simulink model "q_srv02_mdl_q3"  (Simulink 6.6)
settings: Solver=ode1  StartTime=0.0  StopTime=0.5  FixedStep=0.002  RelTol=1e-3  AbsTol=1e-6
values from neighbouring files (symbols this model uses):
  K = Am / Beq_v    [d_model_param.m]    (also in setup_srv02_exp01_mdl.m = 1)
  K_ENC = 0    [config_srv02.m]
  K_POT = -(352 * pi / 180 / 10)    (= -0.614355896702)    [config_srv02.m]
  K_TACH = -(1000 * 2 * pi / 60 / 1.5 / Kg)    [config_srv02.m]
  VMAX_DAC = 10    [setup_srv02_exp01_mdl.m]    (also in setup_srv02_exp02_pos.m; setup_srv02_exp03_spd.m)
  wcf_e = 2 * pi * 25.0    (= 157.079632679)    [setup_srv02_exp01_mdl.m]    (also in setup_srv02_exp02_pos.m = 314.159265359; setup_srv02_exp03_spd.m = 395.840674352)
  zetaf_e = 0.9    [setup_srv02_exp01_mdl.m]    (also in setup_srv02_exp02_pos.m; setup_srv02_exp03_spd.m)
undefined symbols (not defined in the file or in its folder): HIL, IMAX_UPM, qc_get_step_size
libraries: quarc_library x5

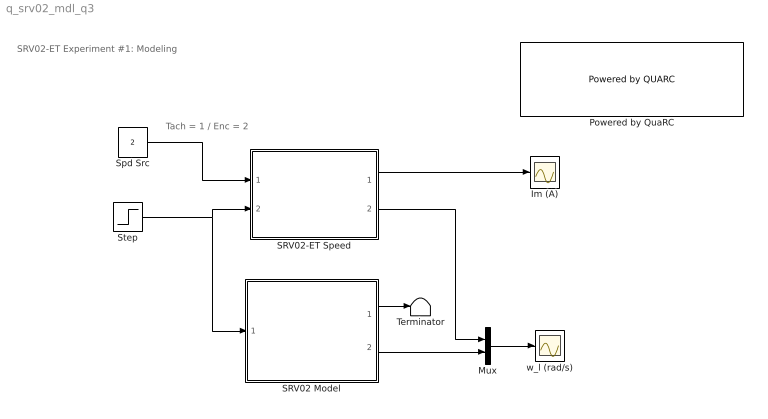
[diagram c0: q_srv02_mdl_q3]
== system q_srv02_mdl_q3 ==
  note: SRV02-ET Experiment #1: Modeling
  note: Tach = 1 / Enc = 2
  Im (A) : Scope
  Mux : Mux  Inputs=2
  Powered by QuaRC : quarc_library/Logos/Powered by QUARC  SystemSampleTime=-1
  SRV02 Model : Subsystem
  SRV02-ET Speed : Subsystem
  Spd Src : Constant  Value=2
  Step : Step  Time=0.1  SampleTime=0
  Terminator : Terminator
  w_l (rad/s) : Scope
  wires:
  Mux/1 -> w_l (rad/s)/1
  SRV02-ET Speed/1(Im (A)) -> Im (A)/1
  SRV02 Model/2(omega_l (rad/s)) -> Mux/2
  SRV02-ET Speed/2(omega_l (rad/s)) -> Mux/1
  SRV02 Model/1(theta_l (rad)) -> Terminator/1
  Spd Src/1 -> SRV02-ET Speed/1(spd src)
  Step/1 -> SRV02-ET Speed/2(I_ref (A)), SRV02 Model/1(I_ref (A))

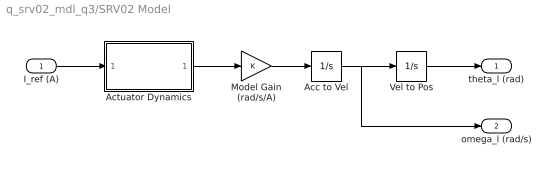
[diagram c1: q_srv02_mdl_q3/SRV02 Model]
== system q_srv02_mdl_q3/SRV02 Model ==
  I_ref (A) : Inport
  Acc to Vel : Integrator
  Actuator Dynamics : Subsystem
  Model Gain (rad/s/A) : Gain  Gain=K
  Vel to Pos : Integrator
  theta_l (rad) : Outport
  omega_l (rad/s) : Outport  Port=2
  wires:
  I_ref (A)/1 -> Actuator Dynamics/1(I_ref (A))
  Acc to Vel/1 -> omega_l (rad/s)/1, Vel to Pos/1
  Actuator Dynamics/1(Im (A)) -> Model Gain (rad/s/A)/1
  Model Gain (rad/s/A)/1 -> Acc to Vel/1
  Vel to Pos/1 -> theta_l (rad)/1

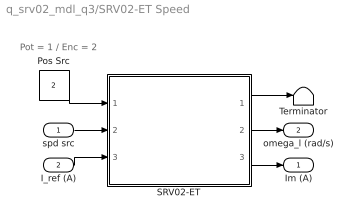
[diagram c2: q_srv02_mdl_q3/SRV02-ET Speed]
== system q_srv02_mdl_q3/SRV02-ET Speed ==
  note: Pot = 1 / Enc = 2
  spd src : Inport
  I_ref (A) : Inport  Port=2
  Pos Src : Constant  Value=2
  SRV02-ET : Subsystem
  Terminator : Terminator
  Im (A) : Outport
  omega_l (rad/s) : Outport  Port=2
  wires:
  SRV02-ET/3(Im (A)) -> Im (A)/1
  I_ref (A)/1 -> SRV02-ET/3(I_ref (A))
  SRV02-ET/2(omega_l (rad/s)) -> omega_l (rad/s)/1
  spd src/1 -> SRV02-ET/2(spd src)
  SRV02-ET/1(theta_l (rad)) -> Terminator/1
  Pos Src/1 -> SRV02-ET/1(pos src)

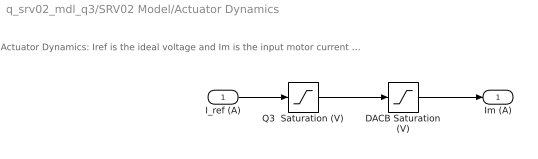
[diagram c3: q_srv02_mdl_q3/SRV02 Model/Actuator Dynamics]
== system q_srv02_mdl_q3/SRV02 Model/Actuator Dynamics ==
  note: Actuator Dynamics: Iref is the ideal voltage and Im is the input motor current after going through the DACB and PWM limitiations.
  I_ref (A) : Inport
  DACB Saturation (V) : Saturate  UpperLimit=VMAX_DAC  LowerLimit=-VMAX_DAC
  Q3  Saturation (V) : Saturate  UpperLimit=IMAX_UPM  LowerLimit=-IMAX_UPM
  Im (A) : Outport
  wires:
  I_ref (A)/1 -> Q3  Saturation (V)/1
  Q3  Saturation (V)/1 -> DACB Saturation (V)/1
  DACB Saturation (V)/1 -> Im (A)/1

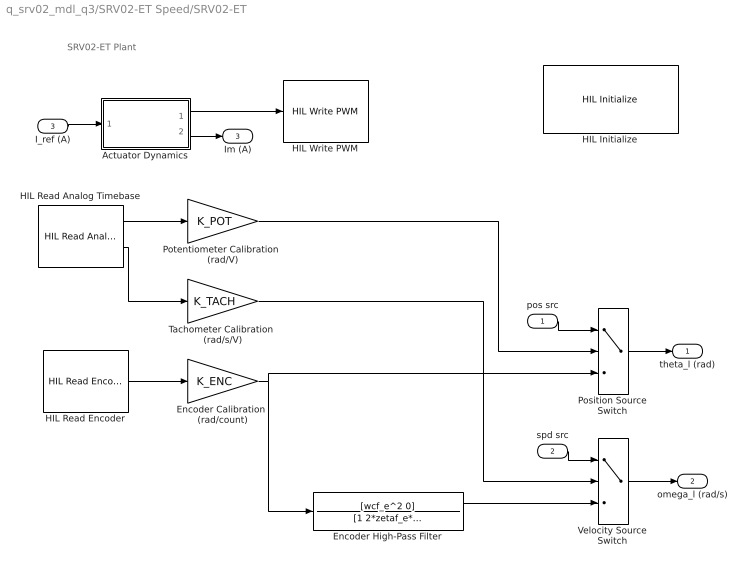
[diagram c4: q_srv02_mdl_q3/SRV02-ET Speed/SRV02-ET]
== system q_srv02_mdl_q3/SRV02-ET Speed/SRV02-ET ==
  note: SRV02-ET Plant
  pos src : Inport
  spd src : Inport  Port=2
  I_ref (A) : Inport  Port=3
  Actuator Dynamics : Subsystem
  Encoder Calibration  (rad/count) : Gain  Gain=K_ENC
  Encoder High-Pass Filter : TransferFcn  Numerator=[wcf_e^2 0]  Denominator=[1 2*zetaf_e*wcf_e wcf_e^2]
  HIL Initialize : quarc_library/Data Acquisition/Generic/Configuration/HIL Initialize  object_name=HIL-1  board_type=q3_controlpaq_fw  board_number=0  exclusive=off  active=on  hardware_clocks=[]  clock_modes=[]  set_clock_params_at_start=off  set_clock_params_at_switch_in=off  analog_input_channels=0:1  analog_input_maximums=10  analog_input_minimums=-10  set_analog_input_params_at_start=off  set_analog_input_params_at_switch_in=off  analog_output_channels=[]  analog_output_maximums=[]  analog_output_minimums=[]  initial_analog_outputs=[]  final_analog_outputs=[]  watchdog_analog_outputs=0  set_analog_output_params_at_start=off  set_analog_output_params_at_switch_in=off  set_analog_outputs_at_start=off  set_analog_outputs_at_switch_in=off  set_analog_outputs_at_terminate=off  set_analog_outputs_at_switch_out=off  set_analog_outputs_on_watchdog=off  digital_input_channels=[]  digital_output_channels=[]  digital_output_configuration=[]  initial_digital_outputs=[]  final_digital_outputs=[]  watchdog_digital_outputs=0  set_digital_output_params_at_start=off  set_digital_output_params_at_switch_in=off  set_digital_outputs_at_start=off  set_digital_outputs_at_switch_in=off  set_digital_outputs_at_terminate=off  set_digital_outputs_at_switch_out=off  set_digital_outputs_on_watchdog=off  encoder_channels=0:2  quadrature=[]  encoder_filter_frequency=[]  initial_encoder_counts=0  set_encoder_params_at_start=off  set_encoder_params_at_switch_in=off  set_encoder_counts_at_start=on  set_encoder_counts_at_switch_in=off  pwm_channels=0:2  pwm_modes=[]  pwm_frequency=[]  pwm_configuration=[]  pwm_alignment=[]  pwm_polarity=[]  pwm_leading_deadband=[]  pwm_trailing_deadband=[]  initial_pwm_outputs=0  final_pwm_outputs=0  watchdog_pwm_outputs=0  set_pwm_params_at_start=off  set_pwm_params_at_switch_in=off  set_pwm_outputs_at_start=on  set_pwm_outputs_at_switch_in=off  set_pwm_outputs_at_terminate=on  set_pwm_outputs_at_switch_out=off  set_pwm_outputs_on_watchdog=off  other_output_channels=[]  initial_other_outputs=[]  final_other_outputs=[]  watchdog_other_outputs=0  set_other_outputs_at_start=off  set_other_outputs_at_switch_in=off  set_other_outputs_at_terminate=off  set_other_outputs_at_switch_out=off  set_other_outputs_on_watchdog=off
  HIL Read Analog Timebase : quarc_library/Data Acquisition/Generic/Timebases/HIL Read Analog Timebase  Tag=unassigned  object_name=HIL-1  clock=0  channels=[0:1]  samples_in_buffer=max(ceil(1/qc_get_step_size), 1)  active=on  vector_output=off
  HIL Read Encoder : quarc_library/Data Acquisition/Generic/Immediate I//O/HIL Read Encoder  Tag=unassigned  object_name=HIL-1  channels=0  sample_time=qc_get_step_size  active=on  vector_output=off  data_type_mode=Inherit via back propagation  data_type=double
  HIL Write PWM : quarc_library/Data Acquisition/Generic/Immediate I//O/HIL Write PWM  object_name=HIL-1  channels=0  sample_time=-1  active=off  vector_input=off
  Position Source Switch : MultiPortSwitch  Inputs=2
  Potentiometer Calibration  (rad/V) : Gain  Gain=K_POT
  Tachometer Calibration  (rad/s/V) : Gain  Gain=K_TACH
  Velocity Source Switch : MultiPortSwitch  Inputs=2
  theta_l (rad) : Outport  InitialOutput=0
  omega_l (rad/s) : Outport  Port=2  InitialOutput=0
  Im (A) : Outport  Port=3  InitialOutput=0
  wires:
  HIL Read Encoder/1 -> Encoder Calibration  (rad/count)/1
  Encoder High-Pass Filter/1 -> Velocity Source Switch/3
  spd src/1 -> Velocity Source Switch/1
  Velocity Source Switch/1 -> omega_l (rad/s)/1
  Actuator Dynamics/2(Im (A)) -> Im (A)/1
  I_ref (A)/1 -> Actuator Dynamics/1(I_ref (A))
  Encoder Calibration  (rad/count)/1 -> Encoder High-Pass Filter/1, Position Source Switch/3
  Tachometer Calibration  (rad/s/V)/1 -> Velocity Source Switch/2
  Actuator Dynamics/1(Vdaq (V)) -> HIL Write PWM/1
  HIL Read Analog Timebase/2 -> Tachometer Calibration  (rad/s/V)/1
  HIL Read Analog Timebase/1 -> Potentiometer Calibration  (rad/V)/1
  pos src/1 -> Position Source Switch/1
  Potentiometer Calibration  (rad/V)/1 -> Position Source Switch/2
  Position Source Switch/1 -> theta_l (rad)/1

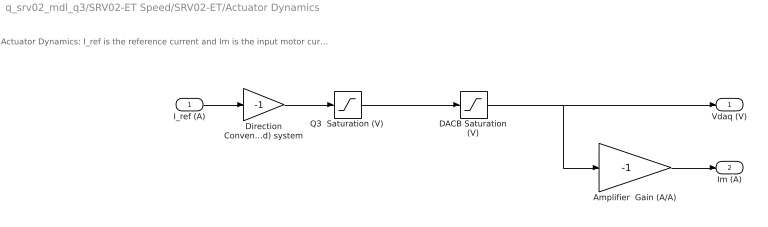
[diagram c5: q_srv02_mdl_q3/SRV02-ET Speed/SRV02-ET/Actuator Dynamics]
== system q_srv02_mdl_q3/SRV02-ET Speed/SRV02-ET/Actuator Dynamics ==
  note: Actuator Dynamics: I_ref is the reference current and Im is the input motor current after going through the DACB and UPM limitiations.
  I_ref (A) : Inport
  Amplifier  Gain (A/A) : Gain  Gain=-1
  DACB Saturation (V) : Saturate  UpperLimit=VMAX_DAC  LowerLimit=-VMAX_DAC
  Direction Convention: (Right-Hand) system : Gain  Gain=-1
  Q3  Saturation (V) : Saturate  UpperLimit=IMAX_UPM  LowerLimit=-IMAX_UPM
  Vdaq (V) : Outport
  Im (A) : Outport  Port=2
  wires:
  Direction Convention: (Right-Hand) system/1 -> Q3  Saturation (V)/1
  Amplifier  Gain (A/A)/1 -> Im (A)/1
  DACB Saturation (V)/1 -> Vdaq (V)/1, Amplifier  Gain (A/A)/1
  Q3  Saturation (V)/1 -> DACB Saturation (V)/1
  I_ref (A)/1 -> Direction Convention: (Right-Hand) system/1
